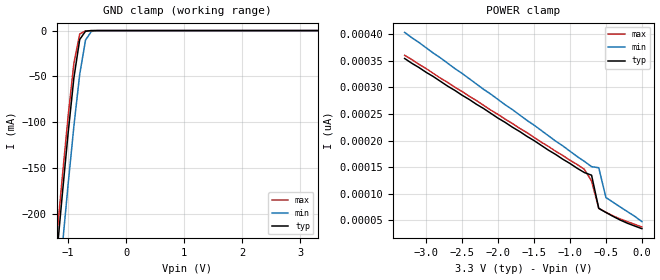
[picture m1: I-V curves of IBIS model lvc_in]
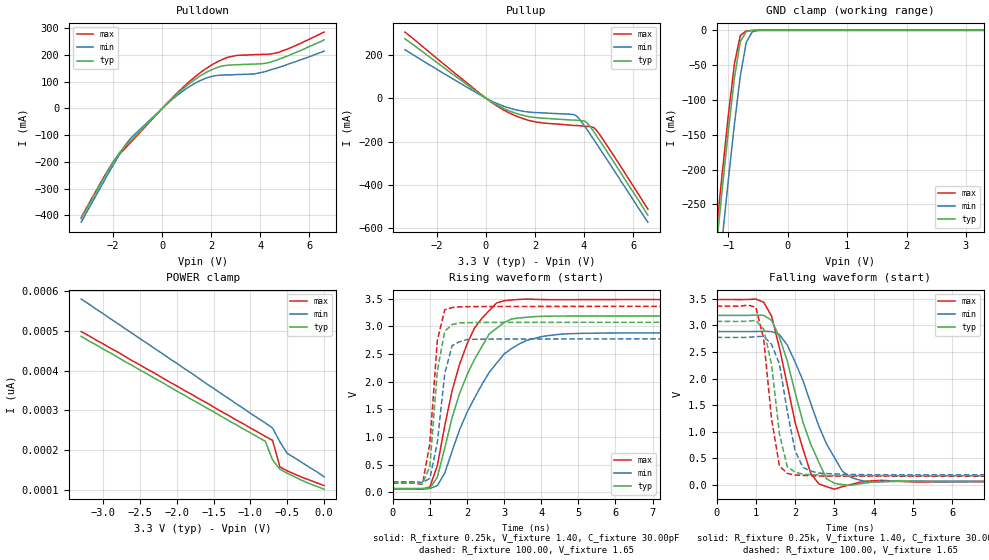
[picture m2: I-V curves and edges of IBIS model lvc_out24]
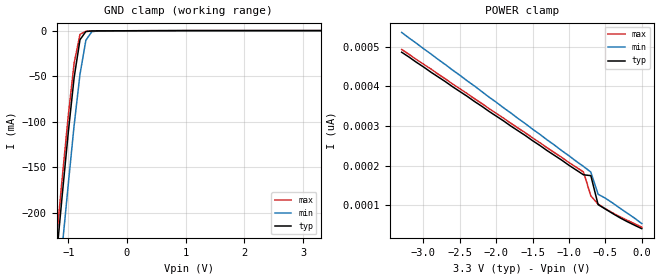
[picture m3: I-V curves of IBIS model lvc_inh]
| IBIS file 16244xh.ibs created by s2ibis2 version 1.1
| North Carolina State University Electronics Research Laboratory  1995
[IBIS ver]   2.1
[File name]   16244xh.ibs
[File Rev]   1.0
[Date]   03/01/99 rtk rtk
[Source]   Integrated Device Technology, Inc.
[Notes]   1.Temperatures: typ=25C, min=100C, max=0C 2.RRmp rates based
   on 50 ohm load.
[Disclaimer] Integrated Device Technology, Inc. ("IDT") hereby grants the
   user of this IBIS model a non-exclusive, nontransferable
   license to use this IBIS model under the following terms. The
   user is granted this license only to use the IBIS model and is
   not granted rights to sell, copy (except as needed to run the
   IBIS model), rent, lease or sub-license the IBIS model in
   whole or in part, or in modified form to anyone. The User may
   modify the IBIS model to suit its specific applications, but
   rights to derivative works and such modifications shall belong
   to IDT. This IBIS model is provided on an AS IS" basis and IDT
   makes absolutely no warranty with respect to the information
   contained herein. IDT DISCLAIMS AND CUSTOMER WAIVES ALL
   WARRANTIES, EXPRESS AND IMPLIED, INCLUDING WARRANTIES OF
   MERCHANTABILITY AND FITNESS FOR A PARTICULAR PURPOSE. THE
   ENTIRE RISK AS TO QUALITY AND PERFORMANCE IS WITH THE USER
   ACCORDINGLY, IN NO EVENT SHALL IDT BE LIABLE FOR ANY DIRECT OR
   INDIRECT DAMAGES, WHETHER IN CONTRACT OR TORT, INCLUDING ANY
   LOST PROFITS OR OTHER INCIDENTAL, CONSEQUENTIAL, EXEMPLARY, OR
   PUNITIVE DAMAGES ARISING OUT OF THE USE OR APPLICATION OF THE
   IBIS model. Further, IDT reserves the right to make changes
   without notice to any product herein to improve reliability,
   function, or design. IDT does not convey any license under
   patent rights or any other intellectual property rights,
   including those of third parties. IDT is not obligated to
   provide maintenance or support for the licensed IBIS model.
[Copyright]   Copyright 1997, Integrated Device Technology, Inc. all rights
   reserved
|   Component LVCH16244
[Component]   LVCH16244
[Manufacturer]   Integrated Device Technology
[Package]
|PA48
| variable   typ   min   max
R_pkg   6.50m   5.00m   10.00m
L_pkg   3.20nH   2.50nH   4.40nH
C_pkg   0.27pF   0.01pF   0.98pF
| PV48   typ   min   max
|R_pkg   6.5m   5.00m   10.00m
|L_pkg   4.75nH   3.82nH   6.72nH
|C_pkg   0.24pF   0.01pF   1.55pF
[Pin]  signal_name   model_name   R_pin   L_pin   C_pin
1   1OEB   lvc_in
2   1Y1   lvc_out24
3   1Y2   lvc_out24
4   GND   GND
5   1Y3   lvc_out24
6   1Y4   lvc_out24
7   VCC   POWER
8   2Y1   lvc_out24
9   2Y2   lvc_out24
10   GND   GND
11   2Y3   lvc_out24
12   2Y4   lvc_out24
13   3Y1   lvc_out24
14   3Y2   lvc_out24
15   GND   GND
16   3Y3   lvc_out24
17   3Y4   lvc_out24
18   VCC   POWER
19   4Y1   lvc_out24
20   4Y2   lvc_out24
21   GND   GND
22   4Y3   lvc_out24
23   4Y4   lvc_out24
24   4OEB   lvc_in
25   3OEB   lvc_in
26   4A4   lvc_inh
27   4A3   lvc_inh
28   GND   GND
29   4A2   lvc_inh
30   4A1   lvc_inh
31   VCC   POWER
32   3A4   lvc_inh
33   3A3   lvc_inh
34   GND   GND
35   3A2   lvc_inh
36   3A1   lvc_inh
37   2A4   lvc_inh
38   2A3   lvc_inh
39   GND   GND
40   2A2   lvc_inh
41   2A1   lvc_inh
42   VCC   POWER
43   1A4   lvc_inh
44   1A3   lvc_inh
45   GND   GND
46   1A2   lvc_inh
47   1A1   lvc_inh
48   2OEB   lvc_in
| Models and submodels in the file (3): lvc_in (Input), lvc_out24 (3-state), lvc_inh (Input)
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| in   in   dummy_model
| oe   oe
|   Model lvc_in
[Model]   lvc_in
Model_type   Input
Vinl =  0.800V
Vinh =  2.000V
C_comp   3.00pF   NA   NA
[Temperature Range]   25.00   100.00   0.000
[Voltage Range]   3.30V   3.00V   3.60V
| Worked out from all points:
|   GND clamp passes 1 mA (typ) near -0.70 V on its own axis
[GND_clamp]
| voltage   I(typ)   I(min)   I(max)
-3.3V     -1.806A    -1.858A    -1.789A
-1.2V     -248mA     -306mA     -229mA
-1.1V     -179mA     -236mA     -160mA
-1V       -112mA     -168mA     -93.56mA
-900mV    -51.39mA   -104mA     -35.36mA
-800mV    -9.697mA   -47.7mA    -3.786mA
-700mV    -714uA     -10.4mA    -348uA
-600mV    -52.42uA   -951uA     -8.225uA
-500mV    -126nA     -30.48uA   -10.89nA
3.3V      34.69pA    75.27pA    23pA
[POWER_clamp]
| voltage   I(typ)   I(min)   I(max)
-3.3V     354pA      403pA      360pA
-800mV    140pA      161pA      146pA
-700mV    135pA      151pA      124pA
-600mV    72.75pA    149pA      72.79pA
-500mV    65.09pA    93.05pA    65.39pA
-300mV    50.77pA    75.27pA    52.78pA
0V        34.68pA    47.91pA    37.83pA
|   Model lvc_out24
[Model]   lvc_out24
Model_type   3-state
Polarity   Non-Inverting
Enable   Active-High
Vinl =  0.000V
Vinh =  2.000V
Vmeas =  1.500V
C_comp   3.00pF   NA   NA
[Temperature Range]   25.00   100.00   0.000
[Voltage Range]   3.30V   3.00V   3.60V
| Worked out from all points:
|   slope of the pulldown table from 0 to 0.495 V, typ, clamps not added: 11.1 ohm
|   slope of the pullup table from 0 to 0.495 V, typ, clamps not added: 14.5 ohm
|   GND clamp passes 1 mA (typ) near -0.65 V on its own axis
|   rising waveform, R_fixture 0.25k, V_fixture 1.40, C_fixture 30.00pF: 20-80 % time 982ps typ, 1.24ns min, 811ps max; typ from 0.061 V to 3.19 V
|   rising waveform, R_fixture 100.00, V_fixture 1.65: 20-80 % time 251ps typ, 304ps min, 220ps max; typ from 0.171 V to 3.08 V
|   falling waveform, R_fixture 0.25k, V_fixture 1.40, C_fixture 30.00pF: 20-80 % time 747ps typ, 915ps min, 646ps max; typ from 3.19 V to 0.061 V
|   falling waveform, R_fixture 100.00, V_fixture 1.65: 20-80 % time 336ps typ, 378ps min, 296ps max; typ from 3.08 V to 0.171 V
[Pulldown]
| voltage   I(typ)   I(min)   I(max)
-3.3V     -413mA     -426mA     -409mA
-2.1V     -217mA     -229mA     -215mA
-1.8V     -173mA     -182mA     -178mA
-1.4V     -132mA     -125mA     -139mA
100mV     9.36mA     8.53mA     9.88mA
900mV     77.5mA     68.6mA     83.2mA
1.8V      135mA      114mA      150mA
2.6V      161mA      126mA      189mA
3.7V      166mA      129mA      201mA
4.4V      173mA      144mA      204mA
5.1V      196mA      165mA      222mA
6.6V      257mA      215mA      286mA
[Pullup]
| voltage   I(typ)   I(min)   I(max)
-3.3V     273mA      223mA      304mA
-200mV    15.7mA     12.6mA     17.8mA
800mV     -51.2mA    -39.9mA    -59.2mA
1.4V      -75.9mA    -58mA      -89.7mA
2V        -89.2mA    -66.1mA    -109mA
3.5V      -101mA     -74.3mA    -125mA
3.7V      -102mA     -83mA      -126mA
4.1V      -112mA     -141mA     -130mA
4.4V      -155mA     -191mA     -136mA
4.5V      -172mA     -208mA     -147mA
5.2V      -292mA     -329mA     -263mA
6.6V      -539mA     -571mA     -511mA
[GND_clamp]
| voltage   I(typ)   I(min)   I(max)
-3.3V     -2.206A    -2.271A    -2.184A
-1.2V     -310mA     -382mA     -286mA
-1.1V     -225mA     -297mA     -202mA
-1V       -144mA     -214mA     -121mA
-900mV    -69.29mA   -136mA     -48.96mA
-800mV    -16.14mA   -65.88mA   -7.431mA
-700mV    -1.8mA     -17.54mA   -933uA
-600mV    -143uA     -2.267mA   -21.88uA
-500mV    -316nA     -75.99uA   -26.99nA
3.3V      101pA      168pA      89pA
[POWER_clamp]
| voltage   I(typ)   I(min)   I(max)
-3.3V     486pA      580pA      498pA
-800mV    222pA      268pA      234pA
-700mV    175pA      255pA      224pA
-600mV    151pA      220pA      157pA
-500mV    141pA      191pA      147pA
-300mV    123pA      168pA      131pA
0V        101pA      132pA      110pA
[Ramp]
| variable   typ   min   max
dV/dt_r   1.45/0.32n   1.21/0.34n   1.64/0.23n
dV/dt_f   1.59/0.39n   1.41/0.50n   1.76/0.35n
R_load = 50.00
[Rising Waveform]
R_fixture = 0.25k
V_fixture = 1.40
C_fixture = 30.00pF
R_dut = 7.00m
L_dut = 3.30nH
C_dut = 0.29pF
| time   V(typ)   V(min)   V(max)
0s        61.33mV    67.59mV    57.9mV
1ns       68.18mV    64.46mV    95.45mV
1.2ns     271mV      118mV      480mV
1.4ns     796mV      346mV      1.199V
1.6ns     1.353V     747mV      1.841V
2ns       2.123V     1.442V     2.681V
2.6ns     2.864V     2.17V      3.286V
3ns       3.069V     2.5V       3.464V
4.6ns     3.186V     2.863V     3.483V
19.8ns    3.189V     2.884V     3.487V
[Rising Waveform]
R_fixture = 100.00
V_fixture = 1.65
R_dut = 7.00m
L_dut = 3.30nH
C_dut = 0.29pF
| time   V(typ)   V(min)   V(max)
0s        171mV      188mV      162mV
600ps     171mV      189mV      159mV
800ps     145mV      174mV      142mV
1ns       470mV      249mV      885mV
1.2ns     2.193V     898mV      2.744V
1.4ns     2.912V     2.145V     3.3V
1.6ns     3.033V     2.652V     3.34V
2ns       3.067V     2.762V     3.356V
2.6ns     3.071V     2.77V      3.359V
19.8ns    3.075V     2.775V     3.362V
[Falling Waveform]
R_fixture = 0.25k
V_fixture = 1.40
C_fixture = 30.00pF
R_dut = 7.00m
L_dut = 3.30nH
C_dut = 0.29pF
| time   V(typ)   V(min)   V(max)
0s        3.189V     2.884V     3.487V
1ns       3.194V     2.885V     3.496V
1.4ns     3.097V     2.883V     3.176V
1.8ns     2.332V     2.631V     1.885V
2.4ns     759mV      1.527V     214mV
2.8ns     115mV      768mV      -35.65mV
3ns       29.9mV     514mV      -81.29mV
3.4ns     -10.27mV   148mV      3.984mV
4ns       54.08mV    51.85mV    76.18mV
19.8ns    61.33mV    67.6mV     57.91mV
[Falling Waveform]
R_fixture = 100.00
V_fixture = 1.65
R_dut = 7.00m
L_dut = 3.30nH
C_dut = 0.29pF
| time   V(typ)   V(min)   V(max)
0s        3.075V     2.775V     3.362V
1ns       3.095V     2.788V     3.342V
1.2ns     2.928V     2.795V     2.746V
1.4ns     2.266V     2.644V     1.244V
1.6ns     960mV      2.279V     356mV
1.8ns     340mV      1.382V     216mV
2ns       239mV      641mV      185mV
2.2ns     199mV      327mV      178mV
2.6ns     183mV      221mV      166mV
19.8ns    171mV      188mV      162mV
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|   Model lvc_inh
[Model]   lvc_inh
Model_type   Input
Vinl =  0.800V
Vinh =  2.000V
C_comp   3.00pF   NA   NA
[Temperature Range]   25.00   100.00   0.000
[Voltage Range]   3.30V   3.00V   3.60V
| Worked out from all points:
|   GND clamp passes 1 mA (typ) near -0.70 V on its own axis
[GND_clamp]
| voltage   I(typ)   I(min)   I(max)
-3.3V     -1.806A    -1.858A    -1.789A
-1.2V     -248mA     -306mA     -229mA
-1.1V     -179mA     -236mA     -160mA
-1V       -112mA     -169mA     -93.63mA
-900mV    -51.47mA   -104mA     -35.47mA
-800mV    -9.82mA    -47.77mA   -3.967mA
-700mV    -887uA     -10.48mA   -557uA
-600mV    -219uA     -1.066mA   -201uA
-500mV    -136uA     -141uA     -155uA
3.3V      163uA      116uA      211uA
[POWER_clamp]
| voltage   I(typ)   I(min)   I(max)
-3.3V     486pA      536pA      493pA
-800mV    177pA      198pA      184pA
-700mV    175pA      184pA      124pA
-600mV    102pA      128pA      103pA
-500mV    90.69pA    118pA      91.59pA
-300mV    68.77pA    93pA       71.38pA
0V        41.28pA    54.13pA    45.03pA
